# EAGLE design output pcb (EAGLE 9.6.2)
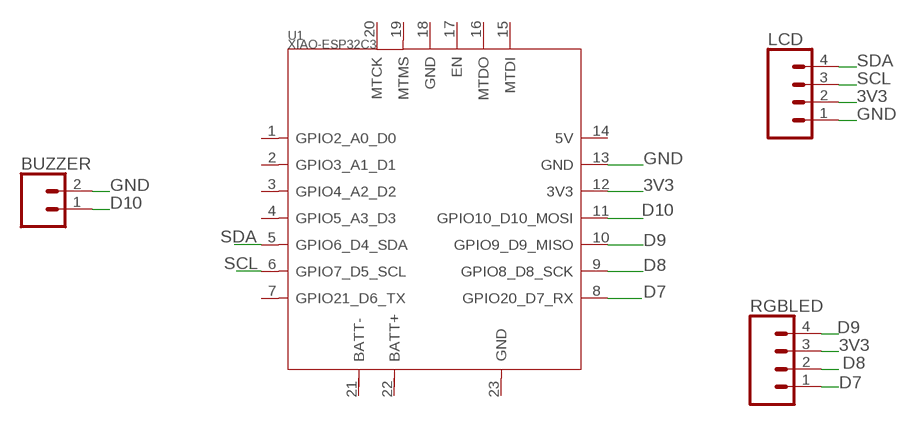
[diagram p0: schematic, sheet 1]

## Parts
BUZZER  CONN_02PAD  [1X02_SOLDER_PADS]
LCD  CONN_04PAD  [1X04_SOLDER_PADS]
RGBLED  CONN_04PAD  [1X04_SOLDER_PADS]
U1  XIAO-ESP32C3  [XIAO-ESP32C3-MODULE14P-2.54-21X17.8MM]

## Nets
3V3: LCD.2 RGBLED.3 U1.12(3V3)
D7: RGBLED.1 U1.8(GPIO20_D7_RX)
D8: RGBLED.2 U1.9(GPIO8_D8_SCK)
D9: RGBLED.4 U1.10(GPIO9_D9_MISO)
D10: BUZZER.1 U1.11(GPIO10_D10_MOSI)
GND: BUZZER.2 LCD.1 U1.13(GND)
SCL: LCD.3 U1.6(GPIO7_D5_SCL)
SDA: LCD.4 U1.5(GPIO6_D4_SDA)
Unconnected: U1.1(GPIO2_A0_D0) U1.2(GPIO3_A1_D1) U1.3(GPIO4_A2_D2) U1.4(GPIO5_A3_D3) U1.7(GPIO21_D6_TX) U1.14(5V) U1.15(MTDI) U1.16(MTDO) U1.17(EN) U1.18(GND) U1.19(MTMS) U1.20(MTCK) U1.21(BATT-) U1.22(BATT+) U1.23(GND)

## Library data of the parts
BUZZER = 2 pin C:CONN_02: Multi connection point. Often used as Generic Header-pin footprint for 0.1 inch spaced/style header connections
LCD RGBLED = 4 pin C:CONN_04: Multi connection point. Often used as Generic Header-pin footprint for 0.1 inch spaced/style header connections On any of the 0.1 inch spaced packages, you can populate with these: Break Away Headers - Straight (PRT-00116) Break Away Male Headers - Right Angle (PRT-00553) Female Headers (PRT-00115)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
U1 = Seeed Studio XIAO Series ESP32 C3:XIAO-ESP32C3: Seeed Studio XIAO ESP32C3 - Espressif ESP32-C3 WiFi BLE Microcontroller - 32-bit 160MHz RISC-V processor Seeed SKU: 113991054 Seeed Studio XIAO ESP32C3 featuring ESP32C3 carries a complete Wi-Fi system along with Bluetooth Low Energy function. With its exquisite design, WiFi+BT ability, it's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

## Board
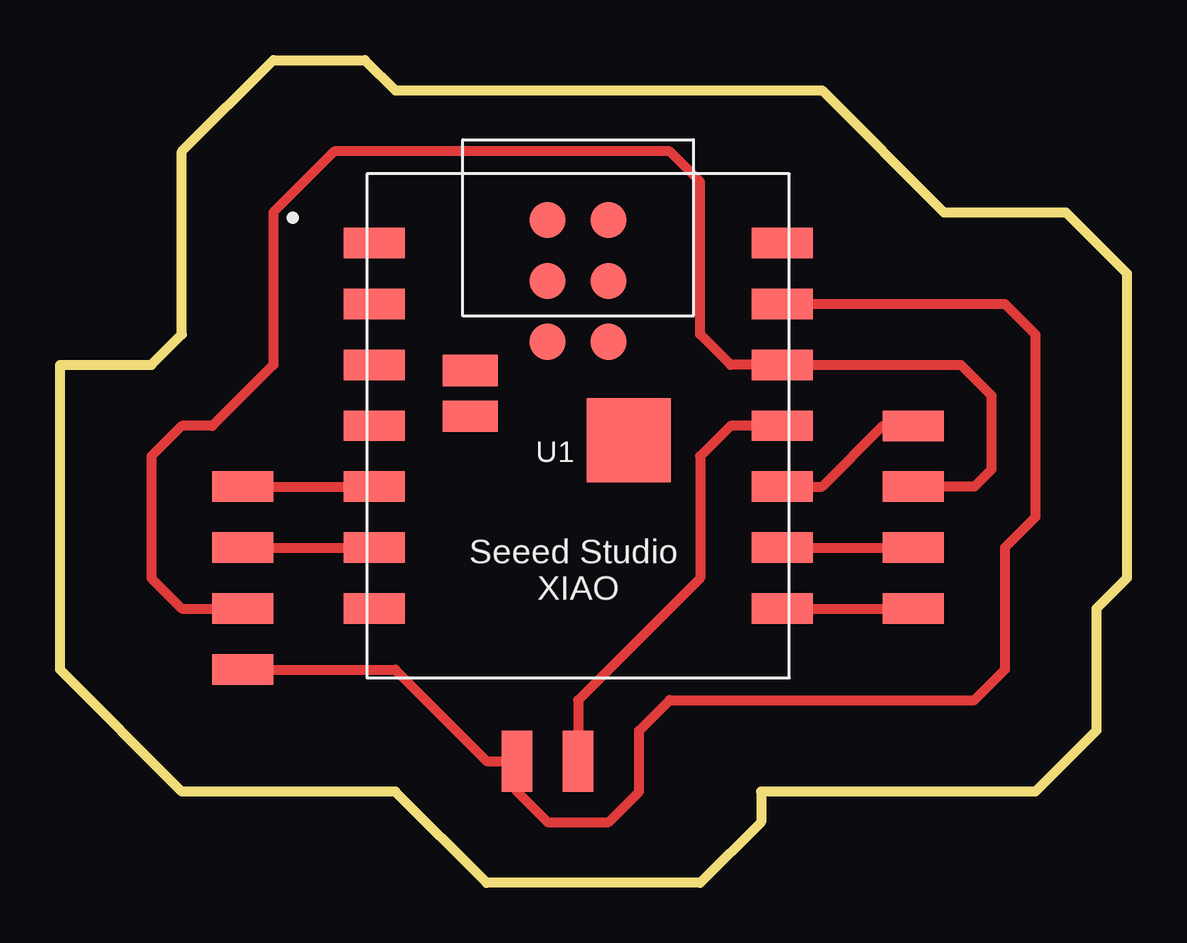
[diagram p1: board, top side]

Size 44.45 x 34.29 mm. Coordinates in mm from the lower left corner, seen from the top.
Outline: 5.08,30.48 8.89,34.29 12.7,34.29 13.97,33.02 31.75,33.02 36.83,27.94 41.91,27.94 44.45,25.4 44.45,12.7 43.18,11.43 43.18,6.35 40.64,3.81 29.21,3.81 29.21,2.54 26.67,0 17.78,0 13.97,3.81 5.08,3.81 0,8.89 0,21.59 3.81,21.59 5.08,22.86 5.08,30.48
Copper layers (1*16): Top 0.035mm / dielectric 0.15mm / Bottom 0.035mm
Design rules "default": minimum track width 6mil, minimum drill 0.35mm, track to track 6mil, track to pad 6mil, pad to pad 6mil, via to via 6mil, smd to smd 6mil, copper to edge 40mil, drill to drill 6mil, minimum pad ring 10mil, minimum via ring 8mil, stop-mask expansion 4mil, vias tented up to drill 0mil, thermal gap 10mil

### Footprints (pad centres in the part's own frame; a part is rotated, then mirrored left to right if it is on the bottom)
1X02_SOLDER_PADS = smd 2.54 x 1.27: 1 0,2.54; 2 0,0
1X04_SOLDER_PADS = smd 2.54 x 1.27: 1 0,2.54; 2 0,5.08; 3 0,7.62; 4 0,10.16
XIAO-ESP32C3-MODULE14P-2.54-21X17.8MM = smd 2.54 x 1.27: 1 -8.5,7.62; 2 -8.5,5.08; 3 -8.5,2.54; 4 -8.5,0; 5 -8.5,-2.54; 6 -8.5,-5.08; 7 -8.5,-7.62; 8 8.5,-7.62; 9 8.5,-5.08; 10 8.5,-2.54; 11 8.5,0; 12 8.5,2.54; 13 8.5,5.08; 14 8.5,7.62 | smd 1.5 x 1.5: 15 -1.27,8.58; 16 1.27,8.58; 17 -1.27,6.04; 18 1.27,6.04; 19 -1.27,3.5; 20 1.27,3.5 | smd 2.3 x 1.3: 21 -4.5,2.3; 22 -4.5,0.4 | smd 3.5 x 3.5: 23 2.1,-0.6

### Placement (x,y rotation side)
BUZZER  19.05,5.08 270 top
LCD  7.62,6.35 0 top
RGBLED  35.56,8.89 0 top
U1  21.59,19.05 0 top

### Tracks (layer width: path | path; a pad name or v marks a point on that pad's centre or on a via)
3V3
  Top 0.406: RGBLED.3 38.1,16.51 38.81,17.22 38.81,20.32 37.54,21.59 U1.12 27.94,21.59 26.67,22.86 26.67,29.21 25.4,30.48 11.43,30.48 8.89,27.94 8.89,21.59 6.35,19.05 5.08,19.05 3.81,17.78 3.81,12.7 5.08,11.43 LCD.2
D7
  Top 0.406: U1.8 RGBLED.1
D8
  Top 0.406: U1.9 RGBLED.2
D9
  Top 0.406: U1.10 31.75,16.51 34.29,19.05 RGBLED.4
D10
  Top 0.406: U1.11 27.94,19.05 26.67,17.78 26.67,12.7 21.59,7.62 BUZZER.1
GND
  Top 0.406: U1.13 39.37,24.13 40.64,22.86 40.64,15.24 39.37,13.97 39.37,8.89 38.1,7.62 25.4,7.62 24.13,6.35 24.13,3.81 22.86,2.54 20.32,2.54 19.05,3.81 BUZZER.2 17.78,5.08 13.97,8.89 LCD.1
SCL
  Top 0.406: LCD.3 U1.6
SDA
  Top 0.406: LCD.4 U1.5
